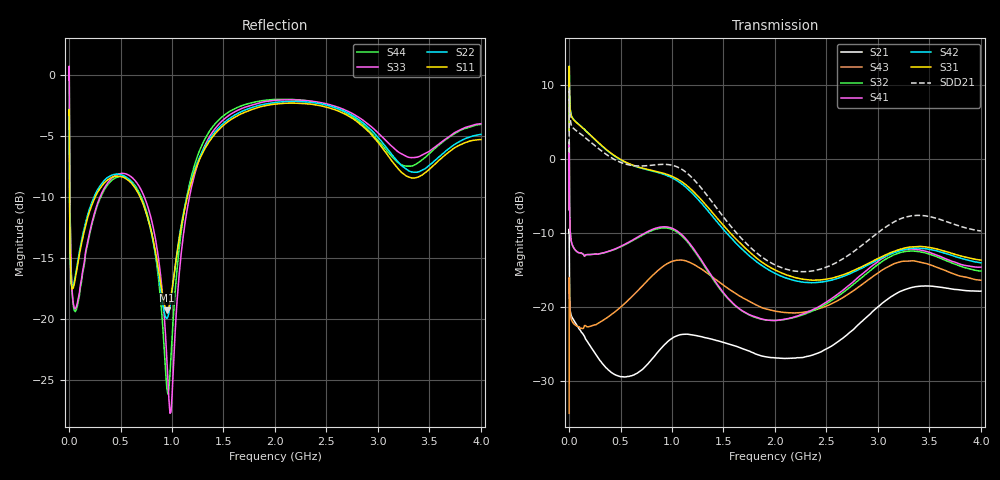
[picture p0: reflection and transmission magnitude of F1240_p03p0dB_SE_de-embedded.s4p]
! Integrated Device Technology
! Corporate Headquarters
! 6024 Silver Creek Valley Road
! San Jose, CA 95138  USA
! Phone:  1-408-284-8200
! Toll Free:  1-800-223-1366
! Webpage:  http://www.idt.com/
! Timing and RF Division
! 515 Groton Road, Suite 102
! Westford, MA 01886-6024
! Device:  F1240
! Description: Dual Intermediate Frequency Digital Variable Gain Amplifier
! Frequency:  10.0 -  500.00 MHz
! Package:  5x5 mm QFN Plastic Package: 32 pin
! Ports:  8 RF, 20 DC
!  Pin  1  = GA3 / Data  Pin 17  = RF OUT_B+
!  Pin  2  = GA4 / CLK  Pin 18  = RF OUT_B-
!  Pin  3  = GA5  Pin 19  = STBY_B
!  Pin  4  = VMODE  Pin 20  = Ground
!  Pin  5  = No Connect  Pin 21  = Ground
!  Pin  6  = GB5  Pin 22  = STB_A
!  Pin  7  = GB4  Pin 23  = RF OUT_A-  = Port 4
!  Pin  8  = GB3  Pin 24  = RF OUT_A+  = Port 3
!  Pin  9  = GB2  Pin 25  = GA0
!  Pin 10  = GB1  Pin 26  = ISET_A
!  Pin 11  = RF IN_B+  Pin 27  = VCC
!  Pin 12  = RF IN_B-  Pin 28  = Ground
!  Pin 13  = Ground  Pin 29  = RF IN_A-  = Port 2
!  Pin 14  = VCC  Pin 30  = RF IN_A+  = Port 1
!  Pin 15  = ISET_B  Pin 31  = GA1
!  Pin 16  = GB0  Pin 32  = GA2 / CSb
! Gain  = +19.5 dB
! State  = 1
! Voltage  = +5.00 V
! Current  = 85.292 mA (one channel only)
! Temperture  =  +25 C
! Test Date  =  2017-10-18
! Board  =  EB4031
! Data:  The device was measured on a custom evaluation board which has
!  individual transmission lines to the RF pins.  Data was collected
!  using a calibrated network analyzer.  The evaluation board was
!  de-embedded using Automatic Fixture Removal.
!  The reference plane is the edge of the package pin.
!  Only Channel A was measured.
!  This data is in single-ended operation.  If your needs are balanced
!  or differential S-parameters then this file needs to be used a
!  linear simulator.
! File Date:  2017-11-10  MJV
! Note:
!  Integrated Device Technology supplies this data as a sample of measured
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# Hz S dB R 100
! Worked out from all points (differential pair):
!   410 points, 500 kHz to 4 GHz, reference 100 ohm
!   strongest paths, dB at 500 kHz, 930 MHz, 1.96 GHz, 2.98 GHz, 4 GHz:
!     S31: 3.8, -2.0, -14.7, -13.6, -13.6
!     S42: 3.8, -2.1, -15.1, -13.8, -14.0
!     S41: -6.9, -9.2, -21.8, -14.1, -14.6
!     S32: -6.8, -9.3, -21.8, -14.5, -15.1
!     S43: -34.3, -14.3, -20.4, -15.6, -16.4
!     S21: -10.0, -25.0, -26.8, -20.2, -17.8
!   taken as a pair (ports 1,2 in; 3,4 out), SDD21 dB: 0.8, -0.7, -14.0, -10.2, -9.7
!   lowest |S11| = -19.3 dB at 950 MHz (marker M1), VSWR 1.24, Z = 81.7 - j7.58 ohm
!   |S11| at or under -10 dB: 4.865 MHz to 253.7 MHz (248.9 MHz wide, 192 % of centre); 691 MHz to 1.148 GHz (457.4 MHz wide, 49.7 % of centre)
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500000  -3.29 -5.5  -9.96 -5.8  -28.88 82.1  -40.63 79.7
        -9.96 -5.7  -3.29 -5.5  -40.59 78.3  -28.87 83.3
        3.84 -105.9  -6.84 -106.5  -0.42 1.2  -34.40 -55.2
        -6.85 -105.4  3.83 -104.8  -34.34 -55.6  -0.43 3.5
2500000  -5.15 -48.5  -13.28 -50.1  -17.94 29.8  -31.52 1.0
         -13.29 -50.0  -5.12 -48.6  -31.49 0.8  -17.94 30.0
         12.01 -178.2  0.60 160.4  -0.89 -52.6  -16.02 -149.4
         0.55 160.5  12.01 -178.0  -16.00 -149.4  -0.95 -52.3
4500000  -9.43 -59.8  -17.97 -43.1  -17.79 13.0  -34.37 -15.3
         -17.97 -43.1  -9.39 -60.0  -34.33 -15.6  -17.79 13.0
         9.45 164.4  -5.09 140.8  -5.01 -77.4  -18.16 179.1
         -5.14 140.9  9.45 164.5  -18.13 179.0  -5.08 -77.3
1.8e8  -11.70 -119.0  -24.67 -52.2  -19.83 -46.9  -36.46 -9.3
       -24.69 -52.1  -11.47 -120.4  -36.51 -8.5  -19.84 -47.2
       3.57 113.7  -12.91 70.4  -13.69 -127.5  -22.74 104.3
       -12.90 70.5  3.57 113.0  -22.66 104.0  -13.83 -126.9
5.2e8  -8.34 -168.1  -29.55 -81.5  -21.28 -110.3  -31.99 -65.8
       -29.40 -80.2  -8.21 -169.7  -32.14 -63.7  -21.43 -110.8
       -0.22 24.8  -11.74 -49.8  -8.05 -168.4  -20.01 11.9
       -11.68 -50.8  -0.26 23.7  -19.77 11.8  -8.31 -168.8
9.5e8  -19.28 -155.1  -24.97 -119.0  -20.19 155.7  -29.28 -154.6
       -24.76 -122.3  -19.93 -153.7  -29.35 -148.4  -20.64 154.3
       -2.08 -82.3  -9.34 175.8  -23.24 160.6  -14.47 -97.8
       -9.17 172.6  -2.23 -84.7  -14.16 -98.3  -25.67 -166.6
4e9  -5.29 -140.7  -17.88 102.3  -24.01 -51.7  -24.91 -34.4
     -17.84 101.9  -4.86 -139.3  -25.73 -18.5  -25.73 -45.5
     -13.65 32.8  -15.13 -74.5  -3.99 -135.5  -17.67 68.6
     -14.61 -88.2  -14.02 38.6  -16.37 58.2  -4.04 -144.9
